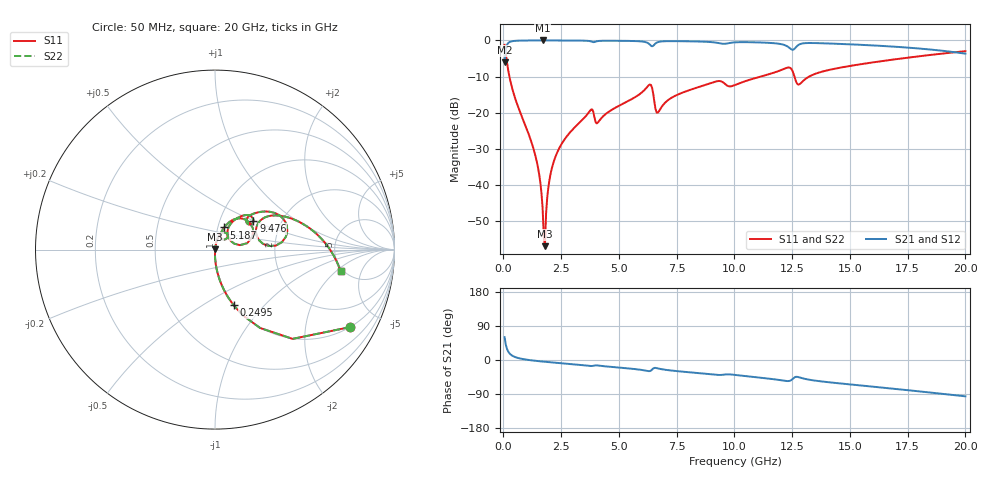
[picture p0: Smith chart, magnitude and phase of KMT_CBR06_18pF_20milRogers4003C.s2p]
! Data measured by Modelithics Inc. support@modelithics.com 813-866-6335
! KEMET CBR0603 18pF, Pad Width= 0.851mm, Pad Length= 0.64mm, Pad Gap= 0.62mm, 20mil Rogers 4003C substrate Data, January 2022
# hz S ma R 50
! 2 Port Network Data from SP1.SP block
! freq  magS11  angS11  magS21  angS21  magS12  angS12  magS22  angS22
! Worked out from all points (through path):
!   401 points, 50 MHz to 20 GHz, reference 50 ohm
!   highest |S21| = -0.01 dB at 1.696 GHz (marker M1); lowest = -6.1 dB at 50 MHz (marker M2)
!   group delay of S21, straight-line fit = 13.6 ps
!   lowest |S11| = -57.0 dB at 1.796 GHz (marker M3), VSWR 1.00, Z = 50.1 + j0.104 ohm
!   |S11| at or under -10 dB: 258.5 MHz to 11.14 GHz (10.89 GHz wide, 191 % of centre); 12.6 GHz to 13.24 GHz (640.1 MHz wide, 4.96 % of centre)
!   |S22| runs from -57.0 to -1.2 dB; largest |S21 - S12| = 0
!   S11 on the Smith chart (normalised r, x): 50 MHz: 0.99, -3.50; 249.5 MHz: 0.99, -0.69; 5.187 GHz: 1.07, +0.27; 9.476 GHz: 1.44, +0.49; 20 GHz: 4.73, -2.31
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5e7  0.8689 -29.8  0.4947 60.2  0.4947 60.2  0.8689 -29.8
2.495e8  0.3263 -71.5  0.9448 18.4  0.9448 18.4  0.3263 -71.5
1.396625e9  0.02426 -90.4  0.9989 -2.2  0.9989 -2.2  0.02426 -90.4
1.596125e9  0.01076 -89.2  0.9991 -3.5  0.9991 -3.5  0.01076 -89.2
1.695875e9  0.004716 -83.8  0.9991 -4.1  0.9991 -4.1  0.004716 -83.8
1.795625e9  0.001411 47.4  0.9991 -4.7  0.9991 -4.7  0.001411 47.4
1.995125e9  0.01186 79.7  0.9989 -5.8  0.9989 -5.8  0.01186 79.7
2.2445e9  0.02416 80.5  0.9986 -7.2  0.9986 -7.2  0.02416 80.5
3.391625e9  0.07802 74.8  0.994 -13.2  0.994 -13.2  0.07802 74.8
3.790625e9  0.1099 60.9  0.969 -15.9  0.969 -15.9  0.1099 60.9
4.089875e9  0.07294 62.0  0.9804 -14.6  0.9804 -14.6  0.07294 62.0
5.187125e9  0.1335 67.5  0.9873 -21.0  0.9873 -21.0  0.1335 67.5
6.33425e9  0.245 37.9  0.8788 -29.3  0.8788 -29.3  0.245 37.9
6.73325e9  0.1045 46.1  0.9575 -22.8  0.9575 -22.8  0.1045 46.1
7.53125e9  0.1768 58.2  0.9768 -29.4  0.9768 -29.4  0.1768 58.2
9.476375e9  0.2665 36.6  0.9004 -39.2  0.9004 -39.2  0.2665 36.6
1.0025e10  0.2412 43.5  0.9408 -39.4  0.9408 -39.4  0.2412 43.5
1.236912e10  0.4214 18.2  0.7946 -55.3  0.7946 -55.3  0.4214 18.2
1.276812e10  0.2446 17.8  0.8642 -45.1  0.8642 -45.1  0.2446 17.8
1.336662e10  0.3315 32.8  0.9208 -53.3  0.9208 -53.3  0.3315 32.8
1.670825e10  0.5343 13.5  0.8277 -74.7  0.8277 -74.7  0.5343 13.5
2e10  0.7101 -9.8  0.6561 -95.9  0.6561 -95.9  0.7101 -9.8
